DATA_BLOCK "IMAC_STANDBY_I/O"
TITLE =
AUTHOR : HottendU
FAMILY : IMAC
VERSION : 0.2


  STRUCT
   STANDBY_001_STAA : WORD ;	//STANDBY - Instance 001 : 'AUTO' Mode  Status  Interface from MOTOR1 A
   STANDBY_001_STAB : WORD ;	//                         'AUTO' Mode  Status  Interface from MOTOR1 B
   STANDBY_001_ACOA : WORD ;	//                         'AUTO' Mode  Command Interface to MOTOR1 A
   STANDBY_001_ACOB : WORD ;	//                         'AUTO' Mode  Command Interface to MOTOR1 B
   STANDBY_001_OSSTAT : WORD ;	//                         OS Status Word
   STANDBY_001_OSALARM : WORD ;	//                         OS Alarm Word
   STANDBY_001_OSCOM : WORD ;	//                         OS Command Interface
   STANDBY_002_STAA : WORD ;	//STANDBY - Instance 002 : 'AUTO' Mode  Status  Interface from MOTOR1 A
   STANDBY_002_STAB : WORD ;	//                         'AUTO' Mode  Status  Interface from MOTOR1 B
   STANDBY_002_ACOA : WORD ;	//                         'AUTO' Mode  Command Interface to MOTOR1 A
   STANDBY_002_ACOB : WORD ;	//                         'AUTO' Mode  Command Interface to MOTOR1 B
   STANDBY_002_OSSTAT : WORD ;	//                         OS Status Word
   STANDBY_002_OSALARM : WORD ;	//                         OS Alarm Word
   STANDBY_002_OSCOM : WORD ;	//                         OS Command Interface
   STANDBY_003_STAA : WORD ;	//STANDBY - Instance 003 : 'AUTO' Mode  Status  Interface from MOTOR1 A
   STANDBY_003_STAB : WORD ;	//                         'AUTO' Mode  Status  Interface from MOTOR1 B
   STANDBY_003_ACOA : WORD ;	//                         'AUTO' Mode  Command Interface to MOTOR1 A
   STANDBY_003_ACOB : WORD ;	//                         'AUTO' Mode  Command Interface to MOTOR1 B
   STANDBY_003_OSSTAT : WORD ;	//                         OS Status Word
   STANDBY_003_OSALARM : WORD ;	//                         OS Alarm Word
   STANDBY_003_OSCOM : WORD ;	//                         OS Command Interface
   STANDBY_004_STAA : WORD ;	//STANDBY - Instance 004 : 'AUTO' Mode  Status  Interface from MOTOR1 A
   STANDBY_004_STAB : WORD ;	//                         'AUTO' Mode  Status  Interface from MOTOR1 B
   STANDBY_004_ACOA : WORD ;	//                         'AUTO' Mode  Command Interface to MOTOR1 A
   STANDBY_004_ACOB : WORD ;	//                         'AUTO' Mode  Command Interface to MOTOR1 B
   STANDBY_004_OSSTAT : WORD ;	//                         OS Status Word
   STANDBY_004_OSALARM : WORD ;	//                         OS Alarm Word
   STANDBY_004_OSCOM : WORD ;	//                         OS Command Interface
   STANDBY_005_STAA : WORD ;	//STANDBY - Instance 005 : 'AUTO' Mode  Status  Interface from MOTOR1 A
   STANDBY_005_STAB : WORD ;	//                         'AUTO' Mode  Status  Interface from MOTOR1 B
   STANDBY_005_ACOA : WORD ;	//                         'AUTO' Mode  Command Interface to MOTOR1 A
   STANDBY_005_ACOB : WORD ;	//                         'AUTO' Mode  Command Interface to MOTOR1 B
   STANDBY_005_OSSTAT : WORD ;	//                         OS Status Word
   STANDBY_005_OSALARM : WORD ;	//                         OS Alarm Word
   STANDBY_005_OSCOM : WORD ;	//                         OS Command Interface
   STANDBY_006_STAA : WORD ;	//STANDBY - Instance 006 : 'AUTO' Mode  Status  Interface from MOTOR1 A
   STANDBY_006_STAB : WORD ;	//                         'AUTO' Mode  Status  Interface from MOTOR1 B
   STANDBY_006_ACOA : WORD ;	//                         'AUTO' Mode  Command Interface to MOTOR1 A
   STANDBY_006_ACOB : WORD ;	//                         'AUTO' Mode  Command Interface to MOTOR1 B
   STANDBY_006_OSSTAT : WORD ;	//                         OS Status Word
   STANDBY_006_OSALARM : WORD ;	//                         OS Alarm Word
   STANDBY_006_OSCOM : WORD ;	//                         OS Command Interface
   STANDBY_007_STAA : WORD ;	//STANDBY - Instance 007 : 'AUTO' Mode  Status  Interface from MOTOR1 A
   STANDBY_007_STAB : WORD ;	//                         'AUTO' Mode  Status  Interface from MOTOR1 B
   STANDBY_007_ACOA : WORD ;	//                         'AUTO' Mode  Command Interface to MOTOR1 A
   STANDBY_007_ACOB : WORD ;	//                         'AUTO' Mode  Command Interface to MOTOR1 B
   STANDBY_007_OSSTAT : WORD ;	//                         OS Status Word
   STANDBY_007_OSALARM : WORD ;	//                         OS Alarm Word
   STANDBY_007_OSCOM : WORD ;	//                         OS Command Interface
   STANDBY_008_STAA : WORD ;	//STANDBY - Instance 008 : 'AUTO' Mode  Status  Interface from MOTOR1 A
   STANDBY_008_STAB : WORD ;	//                         'AUTO' Mode  Status  Interface from MOTOR1 B
   STANDBY_008_ACOA : WORD ;	//                         'AUTO' Mode  Command Interface to MOTOR1 A
   STANDBY_008_ACOB : WORD ;	//                         'AUTO' Mode  Command Interface to MOTOR1 B
   STANDBY_008_OSSTAT : WORD ;	//                         OS Status Word
   STANDBY_008_OSALARM : WORD ;	//                         OS Alarm Word
   STANDBY_008_OSCOM : WORD ;	//                         OS Command Interface
   STANDBY_009_STAA : WORD ;	//STANDBY - Instance 009 : 'AUTO' Mode  Status  Interface from MOTOR1 A
   STANDBY_009_STAB : WORD ;	//                         'AUTO' Mode  Status  Interface from MOTOR1 B
   STANDBY_009_ACOA : WORD ;	//                         'AUTO' Mode  Command Interface to MOTOR1 A
   STANDBY_009_ACOB : WORD ;	//                         'AUTO' Mode  Command Interface to MOTOR1 B
   STANDBY_009_OSSTAT : WORD ;	//                         OS Status Word
   STANDBY_009_OSALARM : WORD ;	//                         OS Alarm Word
   STANDBY_009_OSCOM : WORD ;	//                         OS Command Interface
   STANDBY_010_STAA : WORD ;	//STANDBY - Instance 010 : 'AUTO' Mode  Status  Interface from MOTOR1 A
   STANDBY_010_STAB : WORD ;	//                         'AUTO' Mode  Status  Interface from MOTOR1 B
   STANDBY_010_ACOA : WORD ;	//                         'AUTO' Mode  Command Interface to MOTOR1 A
   STANDBY_010_ACOB : WORD ;	//                         'AUTO' Mode  Command Interface to MOTOR1 B
   STANDBY_010_OSSTAT : WORD ;	//                         OS Status Word
   STANDBY_010_OSALARM : WORD ;	//                         OS Alarm Word
   STANDBY_010_OSCOM : WORD ;	//                         OS Command Interface
  END_STRUCT ;
BEGIN
   STANDBY_001_STAA := W#16#0;
   STANDBY_001_STAB := W#16#0;
   STANDBY_001_ACOA := W#16#0;
   STANDBY_001_ACOB := W#16#0;
   STANDBY_001_OSSTAT := W#16#0;
   STANDBY_001_OSALARM := W#16#0;
   STANDBY_001_OSCOM := W#16#0;
   STANDBY_002_STAA := W#16#0;
   STANDBY_002_STAB := W#16#0;
   STANDBY_002_ACOA := W#16#0;
   STANDBY_002_ACOB := W#16#0;
   STANDBY_002_OSSTAT := W#16#0;
   STANDBY_002_OSALARM := W#16#0;
   STANDBY_002_OSCOM := W#16#0;
   STANDBY_003_STAA := W#16#0;
   STANDBY_003_STAB := W#16#0;
   STANDBY_003_ACOA := W#16#0;
   STANDBY_003_ACOB := W#16#0;
   STANDBY_003_OSSTAT := W#16#0;
   STANDBY_003_OSALARM := W#16#0;
   STANDBY_003_OSCOM := W#16#0;
   STANDBY_004_STAA := W#16#0;
   STANDBY_004_STAB := W#16#0;
   STANDBY_004_ACOA := W#16#0;
   STANDBY_004_ACOB := W#16#0;
   STANDBY_004_OSSTAT := W#16#0;
   STANDBY_004_OSALARM := W#16#0;
   STANDBY_004_OSCOM := W#16#0;
   STANDBY_005_STAA := W#16#0;
   STANDBY_005_STAB := W#16#0;
   STANDBY_005_ACOA := W#16#0;
   STANDBY_005_ACOB := W#16#0;
   STANDBY_005_OSSTAT := W#16#0;
   STANDBY_005_OSALARM := W#16#0;
   STANDBY_005_OSCOM := W#16#0;
   STANDBY_006_STAA := W#16#0;
   STANDBY_006_STAB := W#16#0;
   STANDBY_006_ACOA := W#16#0;
   STANDBY_006_ACOB := W#16#0;
   STANDBY_006_OSSTAT := W#16#0;
   STANDBY_006_OSALARM := W#16#0;
   STANDBY_006_OSCOM := W#16#0;
   STANDBY_007_STAA := W#16#0;
   STANDBY_007_STAB := W#16#0;
   STANDBY_007_ACOA := W#16#0;
   STANDBY_007_ACOB := W#16#0;
   STANDBY_007_OSSTAT := W#16#0;
   STANDBY_007_OSALARM := W#16#0;
   STANDBY_007_OSCOM := W#16#0;
   STANDBY_008_STAA := W#16#0;
   STANDBY_008_STAB := W#16#0;
   STANDBY_008_ACOA := W#16#0;
   STANDBY_008_ACOB := W#16#0;
   STANDBY_008_OSSTAT := W#16#0;
   STANDBY_008_OSALARM := W#16#0;
   STANDBY_008_OSCOM := W#16#0;
   STANDBY_009_STAA := W#16#0;
   STANDBY_009_STAB := W#16#0;
   STANDBY_009_ACOA := W#16#0;
   STANDBY_009_ACOB := W#16#0;
   STANDBY_009_OSSTAT := W#16#0;
   STANDBY_009_OSALARM := W#16#0;
   STANDBY_009_OSCOM := W#16#0;
   STANDBY_010_STAA := W#16#0;
   STANDBY_010_STAB := W#16#0;
   STANDBY_010_ACOA := W#16#0;
   STANDBY_010_ACOB := W#16#0;
   STANDBY_010_OSSTAT := W#16#0;
   STANDBY_010_OSALARM := W#16#0;
   STANDBY_010_OSCOM := W#16#0;
END_DATA_BLOCK

